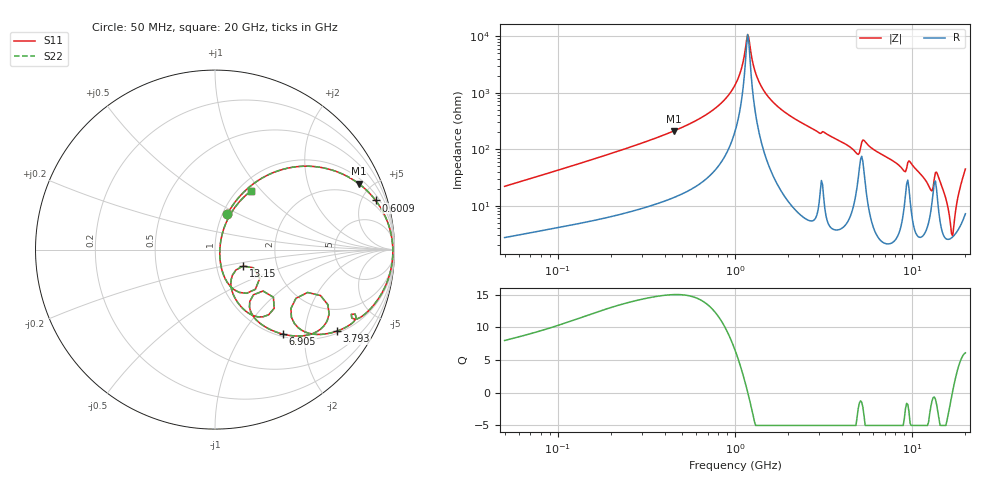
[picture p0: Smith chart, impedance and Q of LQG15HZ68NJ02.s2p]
!Murata Part Number: LQG15HZ68NJ02
!These Parameters are Measured in Series Mode Connection
!  o--[Z]--o
!Port1  Port2
!  o-------o
!Freq. Start=50[MHz] Stop=20[GHz], 401[Steps]
# Hz S RI R 50
!Freq.(Hz) S11(Real) S11(Imag) S21(Real) S21(Imag) S12(Real) S12(Imag) S22(Real) S22(Imag)
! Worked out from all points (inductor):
!   401 points, 50 MHz to 20 GHz, reference 50 ohm
!   read as one part in series: L = 68.4 nH near 51.52 MHz
!   highest Q = 15 at 452.1 MHz (marker M1), where L = 73.9 nH
!   self-resonance near 1.179 GHz
!   S11 on the Smith chart (normalised r, x): 50 MHz: 1.05, +0.44; 600.9 MHz: 1.44, +6.37; 3.793 GHz: 1.07, -2.93; 6.905 GHz: 1.04, -1.55; 13.15 GHz: 1.34, -0.25; 20 GHz: 1.14, +0.88
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5e7  0.0688 0.1982  0.9312 -0.1982  0.9312 -0.1982  0.0688 0.1982
1.364002e8  0.2655 0.4004  0.7345 -0.4004  0.7345 -0.4004  0.2655 0.4004
3.721004e8  0.7186 0.4171  0.2814 -0.4171  0.2814 -0.4171  0.7186 0.4171
4.520922e8  0.8002 0.3679  0.1998 -0.3679  0.1998 -0.3679  0.8002 0.3679
6.009314e8  0.8951 0.274  0.1049 -0.274  0.1049 -0.274  0.8951 0.274
1e9  0.9839 0.0708  0.0161 -0.0708  0.0161 -0.0708  0.9839 0.0708
1.179116e9  0.9908 0.000853  0.00924 -0.000853  0.00924 -0.000853  0.9908 0.000853
1.329223e9  0.9891 -0.0507  0.0109 0.0507  0.0109 0.0507  0.9891 -0.0507
1.521052e9  0.9803 -0.1092  0.0197 0.1092  0.0197 0.1092  0.9803 -0.1092
2.728004e9  0.8371 -0.3579  0.1629 0.3579  0.1629 0.3579  0.8371 -0.3579
3.792786e9  0.6784 -0.4545  0.3216 0.4545  0.3216 0.4545  0.6784 -0.4545
5.117541e9  0.5158 -0.2389  0.4842 0.2389  0.4842 0.2389  0.5158 -0.2389
5.433528e9  0.6246 -0.3981  0.3754 0.3981  0.3754 0.3981  0.6246 -0.3981
6.905011e9  0.3785 -0.4709  0.6215 0.4709  0.6215 0.4709  0.3785 -0.4709
7.442007e9  0.3203 -0.4512  0.6797 0.4512  0.6797 0.4512  0.3203 -0.4512
9.041845e9  0.1938 -0.2885  0.8062 0.2885  0.8062 0.2885  0.1938 -0.2885
1.004137e10  0.238 -0.3744  0.762 0.3744  0.762 0.3744  0.238 -0.3744
1.314879e10  0.1558 -0.0917  0.8442 0.0917  0.8442 0.0917  0.1558 -0.0917
1.417136e10  0.1354 -0.2385  0.8646 0.2385  0.8646 0.2385  0.1354 -0.2385
1.696185e10  0.0274 0.00733  0.9726 -0.00733  0.9726 -0.00733  0.0274 0.00733
1.855685e10  0.0709 0.1693  0.9291 -0.1693  0.9291 -0.1693  0.0709 0.1693
2e10  0.2021 0.328  0.7979 -0.328  0.7979 -0.328  0.2021 0.328
